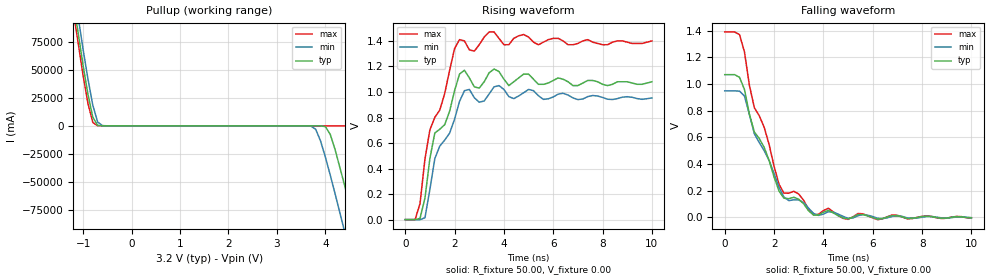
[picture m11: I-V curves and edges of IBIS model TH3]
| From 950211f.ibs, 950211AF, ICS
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|   Model TH3
[Model]   TH3
Model_type   Open_source
Polarity   Inverting
|Vinl = 800.00mV
|Vinh =   2.00V
C_comp   5.50pF   5.00pF   6.00pF
[Temperature Range]   27.00   70.00   0.00
[Voltage Range]   3.20V   3.00V   3.70V
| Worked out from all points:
|   slope of the pullup table from 0 to 0.48 V, typ, clamps not added: 44.7 ohm
|   rising waveform, R_fixture 50.00, V_fixture 0.00: 20-80 % time 988ps typ, 997ps min, 1.06ns max; typ from 0 V to 1.08 V
|   falling waveform, R_fixture 50.00, V_fixture 0.00: 20-80 % time 1.26ns typ, 1.28ns min, 1.26ns max; typ from 1.07 V to -0.004 V
[Pullup]
| voltage   I(typ)   I(min)   I(max)
-3.2V     712.2A     725.6A     703.9A
-1.4V     168.3A     182.8A     159.3A
-1V       53.97A     68.3A      45.07A
-800mV    7.78A      18.54A     3.05A
-700mV    435.7mA    3.38A      89.26mA
3.7V      -21.85mA   -201.2mA   -28.32mA
3.9V      -40.61mA   -13.45A    -28.36mA
4.1V      -7.59A     -43.93A    -28.4mA
4.4V      -53.65A    -95.14A    -33mA
4.6V      -88.23A    -130.3A    -4.43A
5.2V      -195.3A    -237.9A    -101.6A
6.2V      -376.9A    -419.6A    -281.9A
[Ramp]
| variable   typ   min   max
dV/dt_r   645.60m/939.35p   571.98m/948.92p   839.40m/936.90p
dV/dt_f   642.09m/1.20n   570.38m/1.20n   834.33m/1.30n
[Rising Waveform]
R_fixture = 50.00
V_fixture = 0.00
V_fixture_min = 0.00
V_fixture_max = 0.00
| time   V(typ)   V(min)   V(max)
0s        0V         0V         0V
400ps     5.82uV     -59.5nV    -6.43uV
600ps     9.94mV     -455.1uV   126.5mV
800ps     169.3mV    14.86mV    475.8mV
1.2ns     679mV      478.6mV    801.4mV
1.6ns     743.7mV    623mV      987.7mV
2.2ns     1.14V      925.4mV    1.41V
3ns       1.03V      919.5mV    1.37V
3.8ns     1.16V      1.05V      1.42V
10ns      1.08V      953.3mV    1.4V
[Falling Waveform]
R_fixture = 50.00
V_fixture = 0.00
V_fixture_min = 0.00
V_fixture_max = 0.00
| time   V(typ)   V(min)   V(max)
0s        1.07V      948.5mV    1.39V
600ps     1.05V      946.3mV    1.37V
800ps     958.2mV    909.3mV    1.24V
1.2ns     640.4mV    627.1mV    822.3mV
1.6ns     523.9mV    499.5mV    674.9mV
2.4ns     143.6mV    152.2mV    181.8mV
3ns       135.9mV    130.3mV    174.9mV
3.6ns     17.09mV    29.84mV    19.49mV
5ns       -11.29mV   -7.69mV    -15.17mV
10ns      -4.14mV    -2.12mV    -5.55mV
